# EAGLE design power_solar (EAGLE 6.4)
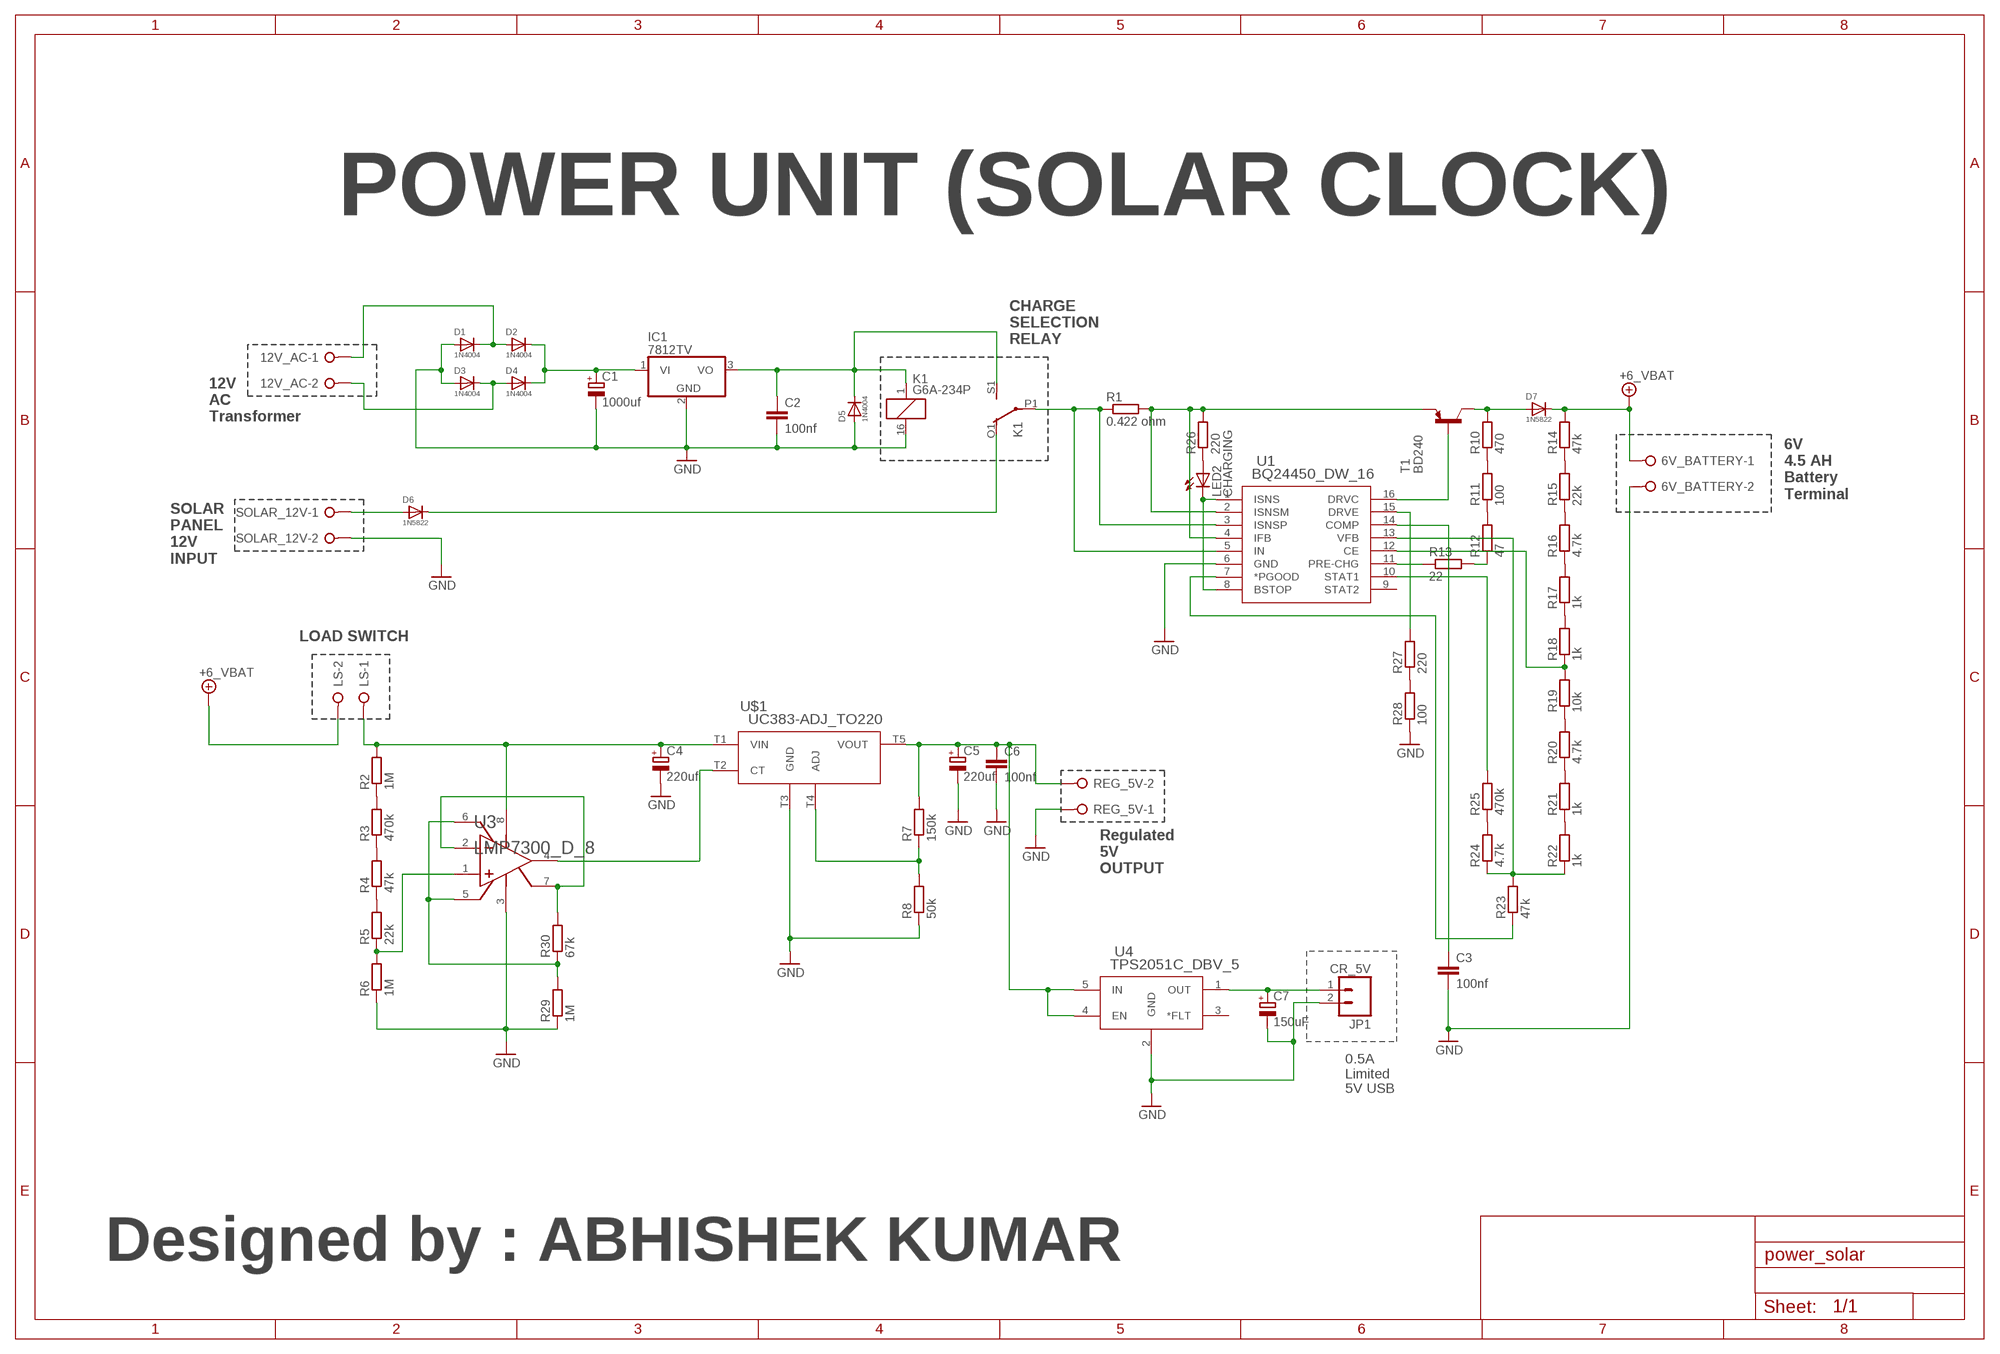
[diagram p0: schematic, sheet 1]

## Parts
6V_BATTERY  W237-02P  [W237-132]
12V_AC  W237-02P  [W237-132]
C1  1000uf  CPOL-EUE3.5-10  [E3,5-10]
C2  100nf  C-EU102-054X133  [C102-054X133]
C3  100nf  C-EU102-054X133  [C102-054X133]
C4  220uf  CPOL-EUE5-8.5  [E5-8,5]
C5  220uf  CPOL-EUE5-8.5  [E5-8,5]
C6  100nf  C-EU050-035X075  [C050-035X075]
C7  150uF  CPOL-EUE2,5-6E  [E2,5-6E]
D1  1N4004  [DO41-10]
D2  1N4004  [DO41-10]
D3  1N4004  [DO41-10]
D4  1N4004  [DO41-10]
D5  1N4004  [DO41-10]
D6  1N5822  DIODE-DO201-15  [DO201-15]
D7  1N5822  DIODE-DO201-15  [DO201-15]
IC1  7812TV  [TO220V]
JP1  CR_5V  M02POLAR  [MOLEX-1X2]
K1  G6A-234P  [G6A-234P]
LED2  CHARGING  LED3MM  [LED3MM]
LS  W237-02P  [W237-132]
R1  0.422 ohm  R-EU_V235/17  [V235/17]
R2  1M  R-EU_R1206  [R1206]
R3  470k  R-EU_R1206  [R1206]
R4  47k  R-EU_R1206  [R1206]
R5  22k  R-EU_R1206  [R1206]
R6  1M  R-EU_R1206  [R1206]
R7  150k  R-EU_R1206  [R1206]
R8  50k  R-EU_R1206  [R1206]
R10  470  R-EU_R1206  [R1206]
R11  100  R-EU_R1206  [R1206]
R12  47  R-EU_R1206  [R1206]
R13  22  R-EU_R1206  [R1206]
R14  47k  R-EU_R1206  [R1206]
R15  22k  R-EU_R1206  [R1206]
R16  4.7k  R-EU_R1206  [R1206]
R17  1k  R-EU_R1206  [R1206]
R18  1k  R-EU_R1206  [R1206]
R19  10k  R-EU_R1206  [R1206]
R20  4.7k  R-EU_R1206  [R1206]
R21  1k  R-EU_R1206  [R1206]
R22  1k  R-EU_R1206  [R1206]
R23  47k  R-EU_R1206  [R1206]
R24  4.7k  R-EU_R1206  [R1206]
R25  470k  R-EU_R1206  [R1206]
R26  220  R-EU_R1206  [R1206]
R27  220  R-EU_R1206  [R1206]
R28  100  R-EU_R1206  [R1206]
R29  1M  R-EU_R1206  [R1206]
R30  67k  R-EU_R1206  [R1206]
REG_5V  W237-02P  [W237-132]
SOLAR_12V  W237-02P  [W237-132]
T1  BD240  BD244  [TO220]
U1  BQ24450_DW_16  [DW16]
U3  LMP7300_D_8  [M08A]
U4  TPS2051C_DBV_5  [DBV5]
U$1  UC383-ADJ_TO220  [TO220-5]

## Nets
GND: 6V_BATTERY.2 C1.- C2.2 C3.2 C4.- C5.- C6.2 C7.- D1.A D3.A D5.A IC1.2(GND) JP1.2 K1.16 R6.1 R8.1 R28.1 R29.1 REG_5V.1 SOLAR_12V.2 U1.6(GND) U3.3(GND) U4.2(GND) U$1.T3(GND)
N$1: C2.1 D5.C IC1.3(VO) K1.1 K1.S1(2:S)
N$2: 12V_AC.2 D3.C D4.A
N$3: 12V_AC.1 D1.C D2.A
N$4: C1.+ D2.C D4.C IC1.1(VI)
N$5: K1.P1(2:P) R1.1 U1.3(ISNSP) U1.5(IN)
N$6: D6.A SOLAR_12V.1
N$7: R1.2 R26.2 T1.3(E) U1.2(ISNSM) U1.4(IFB)
N$8: D6.C K1.O1(2:O)
N$9: T1.1(B) U1.16(DRVC)
N$10: C3.1 U1.14(COMP)
N$11: LED2.K(C) U1.1(ISNS) U1.8(BSTOP)
N$12: D7.A R10.2 T1.2(C)
N$13: C4.+ LS.1 R2.2 U3.8(V+) U$1.T1(VIN)
N$14: R2.1 R3.2
N$15: R3.1 R4.2
N$16: R4.1 R5.2
N$17: R5.1 R6.2 U3.1(IN+)
N$18: U3.4(OUT) U$1.T2(CT)
N$19: R30.2 U3.2(IN-) U3.7(REF)
N$21: C5.+ C6.1 R7.2 REG_5V.2 U4.4(EN) U4.5(IN) U$1.T5(VOUT)
N$22: R7.1 R8.2 U$1.T4(ADJ)
N$24: R10.1 R11.2
N$25: R11.1 R12.2
N$26: R12.1 R13.2
N$27: R13.1 U1.11(PRE-CHG)
N$28: R14.1 R15.2
N$29: R15.1 R16.2
N$30: R16.1 R17.2
N$31: R17.1 R18.2
N$32: R18.1 R19.2 U1.12(CE)
N$33: R19.1 R20.2
N$34: R20.1 R21.2
N$35: R21.1 R22.2
N$36: R22.1 R23.2 R24.1 U1.13(VFB)
N$37: R23.1 U1.7(*PGOOD)
N$38: R24.2 R25.1
N$39: R25.2 U1.10(STAT1)
N$40: LED2.A R26.1
N$41: R27.1 R28.2
N$42: R27.2 U1.15(DRVE)
N$43: C7.+ JP1.1 U4.1(OUT)
N$45: R29.2 R30.1 U3.5(HYSTN) U3.6(HYSTP)
VBAT: 6V_BATTERY.1 D7.C LS.2 R14.2 ; supply symbol labelled +6_VBAT
Unconnected: K1.O2(3:O) K1.P2(3:P) K1.S2(3:S) U1.9(STAT2) U4.3(*FLT)

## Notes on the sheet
- POWER UNIT (SOLAR CLOCK)
- CHARGE
  SELECTION
  RELAY
- 12V
  AC
  Transformer
- 6V
  4.5 AH
  Battery
  Terminal
- SOLAR
  PANEL
  12V
  INPUT
- LOAD SWITCH
- Regulated
  5V
  OUTPUT
- 0.5A
  Limited
  5V USB
- Designed by : ABHISHEK KUMAR

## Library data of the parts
6V_BATTERY 12V_AC LS REG_5V SOLAR_12V = con-wago-508:W237-02P: WAGO SREW CLAMP; OC_FARNELL: unknown; OC_NEWARK: unknown
C1 C4 C5 C7 = resistor:CPOL-EU: POLARIZED CAPACITOR, European symbol
C2 C3 C6 = resistor:C-EU: CAPACITOR, European symbol
D1-D5 = diode:1N4004: DIODE
D6 D7 = diode:DIODE-: DIODE
IC1 = linear:78*: Positive VOLTAGE REGULATOR Source: http://cache.national.com/ds/LM/LM78L05.pdf http://www.fairchildsemi.com/ds/LM/LM7805.pdf
JP1 = SparkFun:M02: Header 2
K1 = relay:G6A-234P: RELAY 2 x switch, 0.3 A/125 V AC, 1 A/30 V DC, Omron; OC_FARNELL: unknown; OC_NEWARK: unknown
LED2 = led:LED: LED
R1-R8 R10-R30 = resistor:R-EU_: RESISTOR, European symbol
T1 = transistor:BD244: PNP TRANSISTOR Source: Motorola Semiconductor, Master Selection Guide Q3/95 SG73 REV 8 page 5.5-5
U1 = BQ24450:BQ24450_DW_16; DATASHEETURL: http://www.ti.com/lit/gpn/BQ24450; DESCRIPTION: Integrated Charge Controller for Lead-Acid Batteries; FAMILY_NAME: BATTERY CHARGE MANAGEMENT; GENERIC_PART_NUMBER: BQ24450; INDUSTRY_STD_PKG_TYPE: SOIC; MANUFACTURER: Texas Instruments; PACKAGE_DESIGNATOR: DW; PIN_COUNT: 16
U3 = LMP7300:LMP7300_D_8
U4 = TPS2051C:TPS2051C_DBV_5; DATASHEETURL: http://www.ti.com/lit/gpn/TPS2051C; DESCRIPTION: Single Channel, Current-Limited USB Power Distribution Switch; FAMILY_NAME: USB POWER SWITCH; GENERIC_PART_NUMBER: TPS2051C; INDUSTRY_STD_PKG_TYPE: SOT-23; MANUFACTURER: Texas Instruments; MANUFACTURER_PART_NUMBER: tps2051c_dbv_5; PACKAGE_DESIGNATOR: DBV; PIN_COUNT: 5; VENDOR: Texas Instruments
U$1 = UCC383-ADJ_KTT_5:UC383-ADJ_TO220

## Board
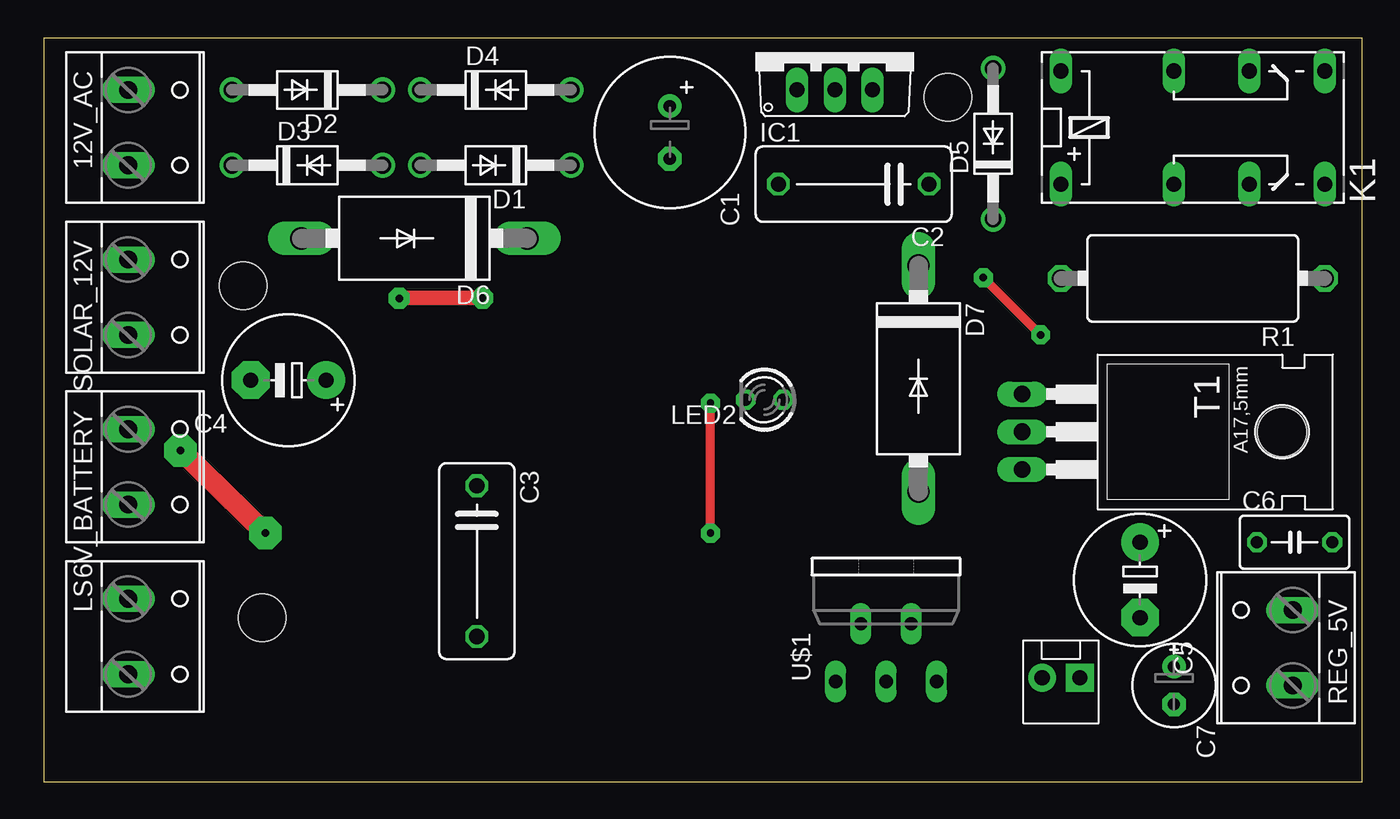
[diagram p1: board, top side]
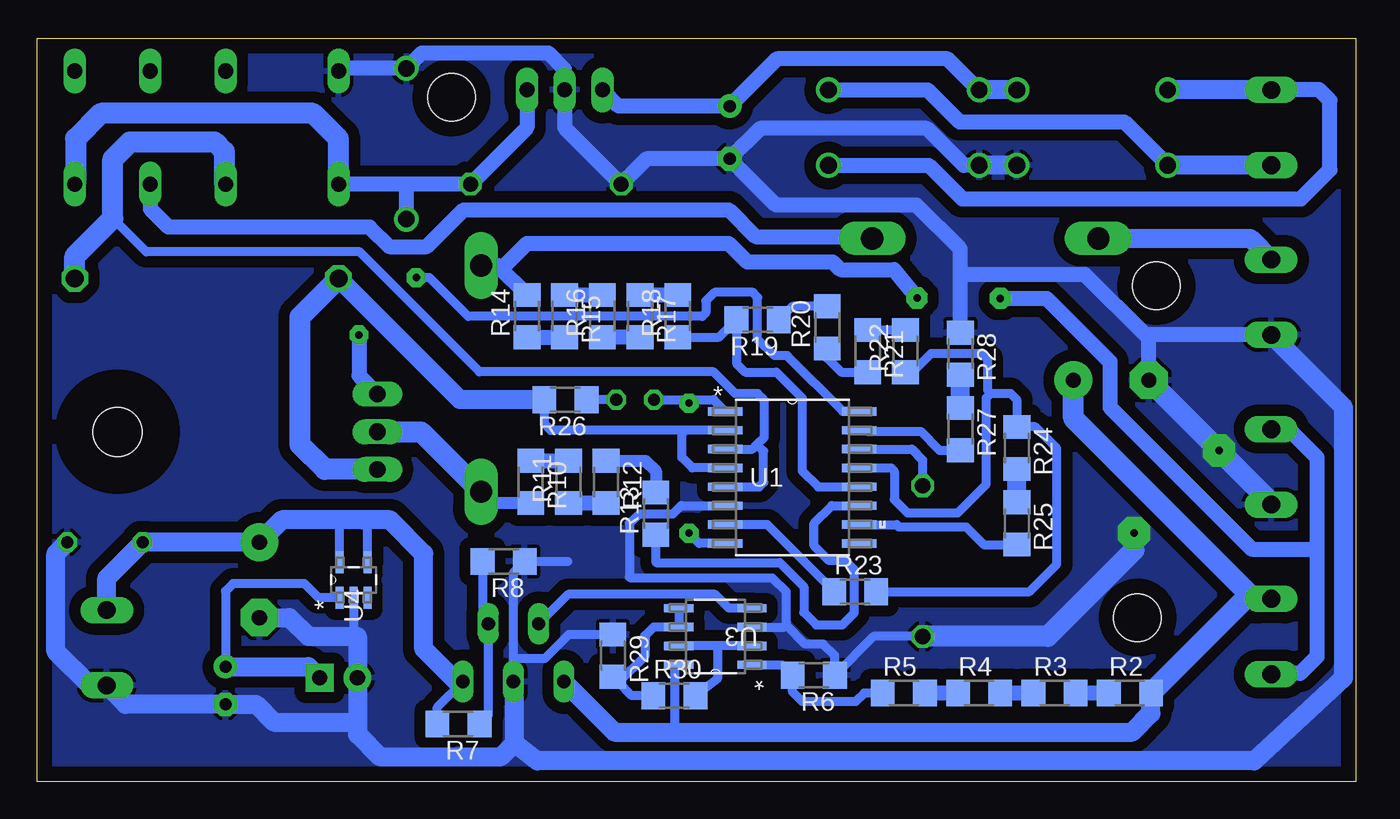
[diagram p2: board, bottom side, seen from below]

Size 88.88 x 50.09 mm. Coordinates in mm from the lower left corner, seen from the top.
Outline: 0,0 88.88,0 88.88,50.09 0,50.09 0,0
Copper layers (1*16): Top 0.035mm / dielectric 1.5mm / Bottom 0.035mm
Design rules "default *": minimum track width 10mil, minimum drill 24mil, track to track 30mil, track to pad 30mil, pad to pad 8mil, via to via 8mil, smd to smd 8mil, copper to edge 40mil, drill to drill 8mil, minimum pad ring 10mil, minimum via ring 8mil, stop-mask expansion 4mil, vias tented up to drill 0mil, thermal gap 10mil
Holes 3.2 mm at 14.73,11.05 60.96,46.1 13.46,33.4

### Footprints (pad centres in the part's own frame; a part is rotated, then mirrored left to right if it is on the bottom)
W237-132 = drill 1.194 long: 1 -2.54,-0.635; 2 2.54,-0.635
E3,5-10 = drill 0.813 pad 1.6: + -1.778,0 | drill 0.813 pad 1.6 octagon: - 1.778,0
C102-054X133 = drill 1.016 octagon: 1 -5.08,0; 2 5.08,0
E5-8,5 = drill 1.016 pad 2.54: + -2.54,0 | drill 1.016 pad 2.54 octagon: - 2.54,0
C050-035X075 = drill 0.813 octagon: 1 -2.54,0; 2 2.54,0
E2,5-6E = drill 0.813 pad 1.575: + -1.27,0 | drill 0.813 pad 1.575 octagon: - 1.27,0
DO41-10 = drill 1.118: A 5.08,0; C -5.08,0
DO201-15 = drill 1.499 long: A 7.62,0; C -7.62,0
TO220V = drill 1.016 long: 1 -2.54,-2.54; 2 0,-2.54; 3 2.54,-2.54
MOLEX-1X2 = drill 1.016 pad 1.88 square: 1 0,0 | drill 1.016 pad 1.88: 2 2.54,0
G6A-234P = drill 1.016 long: 1 -3.81,-3.81; 16 -3.81,3.81; O1 8.89,-3.81; O2 8.89,3.81; P1 3.81,-3.81; P2 3.81,3.81; S1 13.97,-3.81; S2 13.97,3.81
LED3MM = drill 0.813 octagon: A -1.27,0; K 1.27,0
V235/17 = drill 1.194 octagon: 1 -8.89,0; 2 8.89,0
R1206 = smd 1.6 x 1.803: 1 -1.422,0; 2 1.422,0
TO220 = drill 1.118 long: 1 -2.54,-6.35; 2 0,-6.35; 3 2.54,-6.35 | hole 3.302: 0,11.176
DW16 = smd 2.311 x 0.559: 1 -4.521,4.445; 2 -4.521,3.175; 3 -4.521,1.905; 4 -4.521,0.635; 5 -4.521,-0.635; 6 -4.521,-1.905; 7 -4.521,-3.175; 8 -4.521,-4.445; 9 4.521,-4.445; 10 4.521,-3.175; 11 4.521,-1.905; 12 4.521,-0.635; 13 4.521,0.635; 14 4.521,1.905; 15 4.521,3.175; 16 4.521,4.445
M08A = smd 1.981 x 0.559: 1 -2.464,1.905; 2 -2.464,0.635; 3 -2.464,-0.635; 4 -2.464,-1.905; 5 2.464,-1.905; 6 2.464,-0.635; 7 2.464,0.635; 8 2.464,1.905
DBV5 = smd 1.473 x 0.559: 1 -1.194,0.94; 2 -1.194,0; 3 -1.194,-0.94; 4 1.194,-0.94; 5 1.194,0.94
TO220-5 = drill 0.9 long: T1 -3.4,-5.86; T2 -1.7,-1.96; T3 0,-5.86; T4 1.7,-1.96; T5 3.4,-5.86

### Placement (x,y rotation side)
6V_BATTERY  6.35,21.21 270 top
12V_AC  6.35,44.07 270 top
C1  42.21,43.74 270 top
C2  54.61,40.26 180 top
C3  29.21,14.86 270 top
C4  16.51,27.05 180 top
C5  73.91,13.59 270 top
C6  84.33,16.13 0 top
C7  76.2,6.48 270 top
D1  30.48,41.53 180 top
D2  17.78,46.61 180 top
D3  17.78,41.53 0 top
D4  30.48,46.61 0 top
D5  64.01,42.98 90 top
D6  24.99,36.6 180 top
D7  58.98,27.15 270 top
IC1  53.34,49.15 0 top
JP1  69.85,6.98 180 top
K1  72.39,44.07 0 top
LED2  48.59,25.73 180 top
LS  6.35,9.78 270 top
R1  77.47,33.91 180 top
R2  15.24,5.97 0 bottom
R3  20.32,5.97 0 bottom
R4  25.4,5.97 0 bottom
R5  30.48,5.97 0 bottom
R6  36.55,7.16 180 bottom
R7  60.5,3.89 180 bottom
R8  57.45,14.83 180 bottom
R10  55.63,20.19 270 bottom
R11  53.09,20.19 90 bottom
R12  50.55,20.19 270 bottom
R13  47.19,18.06 90 bottom
R14  55.88,31.37 90 bottom
R15  53.34,31.37 270 bottom
R16  50.8,31.37 90 bottom
R17  48.26,31.37 270 bottom
R18  45.72,31.37 90 bottom
R19  40.34,31.11 180 bottom
R20  35.64,30.61 90 bottom
R21  32.92,29.01 270 bottom
R22  30.38,29.01 90 bottom
R23  33.76,12.8 0 bottom
R24  22.86,22.48 270 bottom
R25  22.86,17.4 270 bottom
R26  53.29,25.73 180 bottom
R27  26.67,23.75 270 bottom
R28  26.67,28.83 270 bottom
R29  50.09,8.48 270 bottom
R30  45.95,5.79 0 bottom
REG_5V  83.57,9.02 90 top
SOLAR_12V  6.35,32.64 270 top
T1  72.31,23.57 270 top
U1  38,20.5 0 bottom
U3  43.18,9.78 180 bottom
U4  67.56,13.59 90 bottom
U$1  56.79,12.6 0 top

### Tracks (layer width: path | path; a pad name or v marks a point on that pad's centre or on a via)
GND  (via drill 0.5 pad 2.18)
  Top 1.422: v14.96,16.74 v9.23,22.31
  Bottom 0.61: U3.3 38.53,10.41 38.4,10.54 | 38.4,10.54 38.4,12.78 39.34,13.72 48.89,13.72 48.97,13.79 48.97,17.42 48.26,18.03 46.05,18.03 45.49,18.59 U1.6 | 38.4,10.54 37.13,9.27 35.92,9.27 35.13,8.48 R6.1 32.51,9.78 C3.2 | U4.2 67.56,9.78 | U$1.T3 56.79,8.23 | 56.79,8.23 56.79,14.07 R8.1 53.11,14.83 | R29.1 53.06,9.91 54.69,8.28 56.74,8.28 56.79,8.23
  Bottom 1.016: D1.A 26.44,41.53 28.93,44.02 40.16,44.02 C1.- | C1.- 47.83,41.96 C2.2 53.34,44.07 IC1.2 53.36,46.63 53.36,48.01 54.46,49.1 62.97,49.1 D5.A 68.4,48.06 K1.16 | 26.67,33.96 26.67,35.89 29.62,38.84 39.09,38.84 C1.- | SOLAR_12V.2 14.2,30.1 | 26.67,33.96 26.47,34.16 18.26,34.16 14.2,30.1 | C4.- 13.97,29.87 14.2,30.1 | R28.1 26.67,33.96 | 6V_BATTERY.2 5.71,18.8
  Bottom 1.27: D3.A D1.A | C5.- 71.88,11.05 70.61,9.78 67.56,9.78 67.31,9.78 JP1.2 67.31,4.34 | C6.2 87.63,15.37 87.63,8.76 85.34,6.48 REG_5V.1 82.93,5.21 C7.- 74.14,5.21 72.95,4.01 67.64,4.01 67.31,4.34 | 67.31,4.34 67.31,3.17 65.81,1.68 57.63,1.68 56.72,2.59 | 56.72,2.59 56.72,6.66 U$1.T3 | SOLAR_12V.2 0.84,25.22 0.84,6.98 6.86,1.4 55.19,1.4 56.72,2.59
  Bottom 1.422: C3.2 20.78,9.78 14.96,15.6 v14.96,16.74 | 5.71,18.8 v9.23,22.31 C4.-
  pour Bottom: 0,50.16 -0.03,0.1 88.87,0.1 88.9,50.16
N$1
  Bottom 1.016: IC1.3 55.88,44.07 C2.1 64.08,40.26 | 64.08,40.26 K1.1 | D5.C 64.01,40.18 64.08,40.26
  Bottom 1.422: K1.1 68.58,43.31 70.31,45.03 84.61,45.03 86.31,43.33 86.31,40.31 K1.S1
N$2
  Bottom 1.016: D4.A 28.88,46.61 26.72,44.45 15.62,44.45 D3.C
  Bottom 1.27: 12V_AC.2 D3.C
N$3
  Bottom 1.016: D1.C 28.8,41.53 26.54,39.27 3.71,39.27 1.75,41.22 1.75,45.9 2.49,46.63 5.69,46.63 12V_AC.1
  Bottom 1.27: 12V_AC.1 D2.A
N$4
  Bottom 1.016: D4.C 25.45,46.61 27.53,48.69 39.04,48.69 C1.+ 49.71,45.52 IC1.1
  Bottom 1.27: D2.C D4.C
N$5
  Bottom 0.61: U1.3 40.69,22.4 40.37,22.72 | 40.37,22.72 39.88,23.22 39.88,25.68 40.33,26.14 41.83,26.14 43.31,27.61 59.08,27.61 67.16,35.69 81.53,35.69 83.8,37.95 | U1.5 40.23,19.86 39.93,20.17 39.93,22.28 40.37,22.72
  Bottom 1.422: R1.1 86.36,35.38 83.8,37.95 83.8,41.94 82.63,43.1 76.94,43.1 76.28,42.44 76.28,40.33 K1.P1
N$6
  Bottom 1.27: D6.A 7.14,36.6 SOLAR_12V.1
N$7
  Bottom 0.61: U1.2 45.19,23.67 | 45.19,23.67 54.28,23.67 54.71,24.11 R26.2 | U1.4 44.73,21.13 45.44,21.84 45.44,23.42 45.19,23.67
  Bottom 1.27: R26.2 60.4,25.73 R1.2
  Bottom 1.422: T1.3 69.49,21.03 71.17,22.71 71.17,31.32 R1.2
N$8
  Bottom 1.016: K1.O1 81.26,40.23 81.26,38.58 80.04,37.36 66.47,37.36 65.15,36.04 62.64,36.04 60.15,38.53 42.27,38.53 40.46,36.73 32.74,36.73 D6.C
N$9  (via drill 0.5 pad 1.27)
  Top 0.61: v63.35,33.96 v67.21,30.1
  Bottom 0.61: U1.16 34.59,24.94 38.35,28.7 39.19,28.7 40.33,29.79 40.33,32.61 40.64,32.97 43.23,32.97 43.81,32.39 43.81,31.6 44.07,31.34 59.84,31.34 62.46,33.96 v63.35,33.96
  Bottom 1.016: v67.21,30.1 67.21,27.36 T1.1
N$10
  Bottom 0.61: U1.14 29.95,22.4 29.21,21.67 C3.1
N$11  (via drill 0.5 pad 1.27)
  Top 0.61: v44.96,16.74 v44.96,25.5
  Bottom 0.61: U1.8 44.27,16.05 v44.96,16.74 | LED2.K 45.19,25.73 | 45.19,25.73 43.31,25.73 U1.1 | v44.96,25.5 45.19,25.73
N$12
  Bottom 0.813: R10.2 58.22,18.77 D7.A
  Bottom 1.422: T1.2 63.02,23.57 D7.A
N$13
  Bottom 0.61: U3.8 45.95,7.87 45.95,3.35 45.97,3.33
  Bottom 1.27: R2.2 13.82,4.6 15.09,3.33 45.97,3.33 49.98,3.33 U$1.T1 | R2.2
  Bottom 1.422: R2.2 7.47,12.32 LS.1 6.88,12.32 19.05,24.49 C4.+
N$14
  Bottom 1.016: R2.1 R3.2
N$15
  Bottom 1.016: R3.1 R4.2
N$16
  Bottom 1.016: R4.1 R5.2
N$17
  Bottom 0.61: U3.1 38.68,7.87 R6.2 37.97,6.05 37.31,5.38 33.73,5.38 33.15,5.97 R5.1
N$18
  Bottom 0.61: U3.4 42.27,11.68 43.2,12.62 53.11,12.62 U$1.T2
N$19
  Bottom 0.61: U3.2 42.93,9.14 | 42.93,9.14 U3.7 | 42.93,9.14 43.05,9.02 43.05,6.93 R30.2
N$21
  Bottom 0.61: U4.4 66.62,17.3 66.95,17.63 | U4.5 68.5,17.6 68.48,17.63 | R7.2 61.92,5.01 U$1.T5
  Bottom 1.27: REG_5V.2 84.2,13.72 C6.1 C5.+ 72.42,17.63 68.48,17.63 66.95,17.63 65.1,17.63 62.84,15.37 62.84,8.94 60.64,6.74 U$1.T5
N$22
  Bottom 0.61: R8.2 58.88,11.02 U$1.T4 58.49,4.47 R7.1
N$24
  Bottom 1.016: R10.1 R11.2
N$25
  Bottom 1.016: R12.2 R11.1
N$26
  Bottom 0.813: R12.1 47.88,21.61 47.19,20.93 R13.2
N$27
  Bottom 0.61: R13.1 47.19,15.39 47.17,14.76 38.84,14.76 37.21,13.13 37.21,11.41 36.37,10.57 34.62,10.57 33.81,11.38 33.81,14.28 34.42,14.88 35.51,14.88 36.52,15.9 36.52,17.4 35.33,18.59 U1.11
N$28
  Bottom 1.016: R14.1 R15.2
N$29
  Bottom 1.016: R15.1 R16.2
N$30
  Bottom 1.016: R17.2 R16.1
N$31
  Bottom 1.016: R17.1 R18.2
N$32
  Bottom 0.61: U1.12 36.25,19.86 37.34,20.95 37.34,25.86 39.06,27.58 41.17,27.58 41.76,28.17 R19.2 42.92,29.95 R18.1
N$33
  Bottom 0.61: R20.2 38,32.03 R19.1
N$34
  Bottom 0.61: R20.1 35.64,28.52 34.7,27.58 R21.2
N$35
  Bottom 0.61: R22.2 R21.1
N$36
  Bottom 0.61: 24.61,26.16 24.84,26.39 24.84,28.47 25.22,28.85 28.63,28.85 30.07,27.41 | 24.61,26.16 24.92,25.86 24.92,20.04 26.85,18.11 30.23,18.11 31.11,19 31.11,20.9 31.34,21.13 U1.13 | 24.61,26.16 23.29,26.16 22.86,25.73 R24.1 | R23.2 22.02,12.8 20.17,14.66 20.17,22.45 21.62,23.9 R24.1 | R24.1 | 30.35,27.13 30.07,27.41 | R22.1 30.25,27.58 30.07,27.41
N$37
  Bottom 0.61: R23.1 35.18,12.83 39.67,17.32 U1.7
N$38
  Bottom 1.27: R25.1 R24.2
N$39
  Bottom 0.61: R25.2 25.09,15.98 26.29,17.17 30.81,17.17 30.96,17.32 U1.10 | R25.2
N$40
  Bottom 0.61: LED2.A R26.1
N$41
  Bottom 1.27: R27.1 R28.2
N$42
  Bottom 0.61: U1.15 32.97,23.67 32.89,23.6 29.34,23.6 28.07,22.33 R27.2 | R27.2
N$43
  Bottom 0.61: U4.1 69.93,12.39 70.87,13.34 75.69,13.34 76.2,12.83 C7.+
  Bottom 1.27: C7.+ 70.61,7.75 JP1.1
N$45
  Bottom 0.61: U3.5 U3.6 47.35,10.41 47.93,9.83 47.93,8.46 49.71,6.68 | R30.1 48.82,5.79 49.71,6.68 | 49.71,6.68 R29.2
VBAT  (via drill 0.5 pad 1.42)
  Top 1.016: v29.59,32.59 v23.98,32.56
  Bottom 1.016: 6V_BATTERY.1 4.55,23.75 2.64,21.84 2.64,15.75 | 2.64,15.75 2.64,8.41 3.76,7.29 5.66,7.29 LS.2 | R14.2 57.86,34.77 D7.C 57.38,34.77 55.88,36.27 42.29,36.27 41.05,35.03 35.28,35.03 34.75,34.49 31.14,34.49 v29.59,32.59 | 2.64,15.75 2.72,15.67 7.04,15.67 16.59,25.22 16.59,28.3 20.85,32.56 v23.98,32.56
